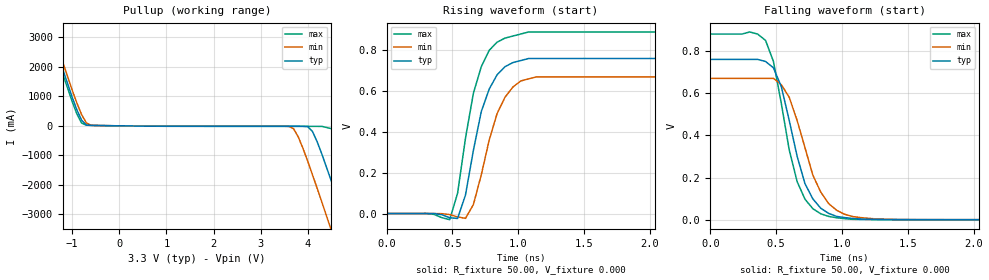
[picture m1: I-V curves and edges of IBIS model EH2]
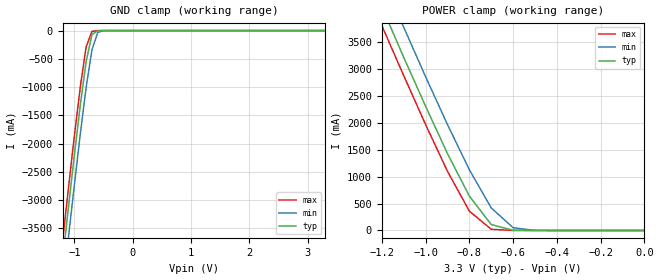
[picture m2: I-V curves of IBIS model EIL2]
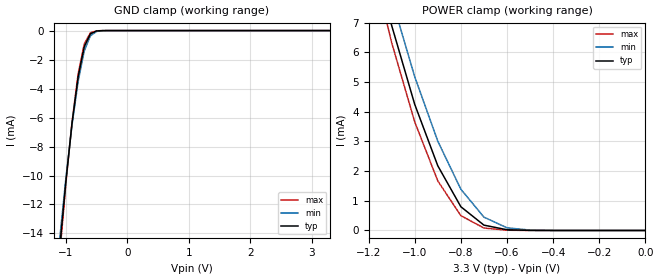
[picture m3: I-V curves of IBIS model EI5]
|   * 932s801a.ibs * IBIS 2.1 Model file
| Rev History
| Rev No.   Description
| 1.0   Initial release with Updated Parasitic Parameters
[IBIS Ver]   2.1
[Comment char]  |_char
[File name]   932s801a.ibs
[Date]   May 19, 2004
[File Rev]   1.0
[Source]   Originated at Integrated Circuit Systems, Inc.
[Disclaimer] (C) Copyright Integrated Circuit Systems, Inc. 2004
   All rights reserved
ICS hereby grants the user of this IBIS model a non-exclusive,
nontransferable license to use this IBIS model under the following terms.
Before using this IBIS model, the user should read this license.
If the user does not accept these terms,  the IBIS model should be
returned to ICS within 30 days.
   The user is granted this license only to use the IBIS model and
is not granted rights to sell, load, rent, lease or license the IBIS
model in whole or in part, or in modified form to anyone other than
user. User may modify the IBIS model to suit its specific
applications but rights to derivative works and such modifications
shall belong to ICS.
   This IBIS model is provided on an "AS IS" basis and ICS makes
absolutely no warranty with respect to the information contained
herein. ICS DISCLAIMS AND CUSTOMER WAIVES ALL WARRANTIES, EXPRESS
OR IMPLIED, INCLUDING WARRANTIES OF MERCHANTABILITY OR FITNESS FOR
A PARTICULAR PURPOSE. The entire risk as to quality and performance
is with the Customer. ACCORDINGLY, IN NO EVENT SHALL THE COMPANY BE
LIABLE FOR ANY DAMAGES, WHETHER IN CONTRACT OR TORT,INCLUDING ANY
LOST PROFITS OR OTHER INCIDENTAL, CONSEQUENTIAL, EXEMPLARY, OR
PUNITIVE DAMAGES ARISING OUT OF THE USE OR APPLICATION OF THE IBIS
model provided in this package. Further, ICS reserves the right to
make changes without notice to any product herein to improve
reliability, function, or design. ICS does not convey any license
under patent rights or any other intellectual property rights,
including those of third parties.
   ICS is not obligated to provide maintenance or support
for the licensed IBIS model.
|   COMPONENT: ICS932s801a
[Component]   ICS932s801a
[Manufacturer]  ICS
[Package]
| variable   typ   min   max
R_pkg   81.1m   62.2m   100.0m
L_pkg   6.7nH   4.9nH   8.5nH
C_pkg   0.53pF  0.21pF  0.85pF
[Pin]   signal_name   model_name   R_pin   L_pin   C_pin
  1   X1   EIX
  2   X2   EIX
  3   VDD48   POWER
  4   M48_0   YO39
  5   M48_1   YO39
  6   GND   GND
  7   SCLK   EI8
  8   SDATA   EIOD1
  9   VDDHTT   POWER
  10   HTTCLK0   FIO2
  11   HTTCLK1   FIO2
  12   HTTCLK2   FIO2
  13   HTTCLK3   FIO2
  14   GND   GND
  15   VDDPCI   POWER
  16   PCI0   FIO2
  17   PCI1   FIO2
  18   PCI2   FIO2
  19   PCI3   FIO2
  20   GND   GND
  21   PDB   EI5
  22   VDDA   POWER
  23   VSSA   GND
  24   IREF   EI5
  25   SRCCLKC0   EH2
  26   SRCCLKT0   EH2
  27   VDDSRC   POWER
  28   GND   GND
  29   SPREAD_EN   EI5
  30   CPU3B   DO10
  31   CPU3   DO10
  32   VSSCPU   GND
  33   VDDCPU   POWER
  34   CPU2B   DO10
  35   CPU2   DO10
  36   VSSCPU   GND
  37   VDDCPU   POWER
  38   CPU1B   DO10
  39   CPU1   DO10
  40   VSSCPU   GND
  41   VDDCPU   POWER
  42   CPU0B   DO10
  43   CPU0   DO10
  44   GND   GND
  45   FS2   EIL2
  46   FS1_REF1   EIO20
  47   FS0_REF0   EIO20
  48   VDDREF   POWER
|* Either 3.3V or 2.5V
|** All model are simulated with typical corner process
[Diff Pin]   inv_pin   vdiff   tdelay_typ
14   15   NA   NA
17   18   NA   NA
21   22   NA   NA
23   24   NA   NA
26   27   NA   NA
31   30   NA   NA
33   32   NA   NA
36   35   NA   NA
42   41   NA   NA
45   44   NA   NA
| Models and submodels in the file (10): EH2 (Open_source), EIL2 (Input), EI5 (Input), EI8 (Input), EIOD1 (I/O_open_drain), EIX (Input), DO10 (Output), FIO2 (I/O), EIO20 (I/O), YO39 (Output)
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|   Model EH2
[Model]   EH2
Model_type   Open_source
Polarity   Inverting
C_comp   5.50pF   5.00pF   6.00pF
[Temperature Range]   27.00   70.00   0.000
[Voltage Range]   3.30V   3.00V   3.70V
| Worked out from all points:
|   slope of the pullup table from 0 to 0.495 V, typ, clamps not added: 56.2 ohm
|   rising waveform, R_fixture 50.00, V_fixture 0.000: 20-80 % time 162ps typ, 178ps min, 159ps max; typ from 0 V to 0.76 V
|   falling waveform, R_fixture 50.00, V_fixture 0.000: 20-80 % time 187ps typ, 213ps min, 169ps max; typ from 0.76 V to 0 V
[Pullup]
| voltage   I(typ)   I(min)   I(max)
-3.3V     12.3A      12.52A     12.16A
-1.7V     4.31A      4.55A      4.16A
-1.5V     3.33A      3.58A      3.17A
-900mV    540mA      770mA      400mA
-700mV    28.62mA    98.17mA    20.44mA
3.7V      -15.27mA   -98.54mA   -17.77mA
4.1V      -190mA     -1.66A     -17.8mA
4.5V      -1.87A     -3.54A     -94.68mA
4.7V      -2.82A     -4.51A     -810mA
4.9V      -3.78A     -5.48A     -1.72A
5.3V      -5.73A     -7.43A     -3.63A
6.6V      -12.13A    -13.84A    -10.01A
[Ramp]
| variable   typ   min   max
dV/dt_r   0.46/0.16n   0.40/0.17n   0.53/0.15n
dV/dt_f   0.45/0.18n   0.40/0.20n   0.53/0.17n
R_load = 50.00
[Rising Waveform]
R_fixture = 50.00
V_fixture = 0.000
V_fixture_min = 0.000
V_fixture_max = 0.000
| time   V(typ)   V(min)   V(max)
0s        0V         0V         0V
480ps     -20.65mV   -5.16mV    -30.15mV
540ps     -24.16mV   -16.59mV   100mV
600ps     91.23mV    -23.49mV   370mV
660ps     310mV      44.3mV     590mV
720ps     500mV      190mV      720mV
840ps     680mV      490mV      840mV
900ps     720mV      570mV      860mV
1.14ns    760mV      670mV      890mV
3ns       760mV      670mV      890mV
[Falling Waveform]
R_fixture = 50.00
V_fixture = 0.000
V_fixture_min = 0.000
V_fixture_max = 0.000
| time   V(typ)   V(min)   V(max)
0s        760mV      670mV      880mV
420ps     750mV      670mV      850mV
480ps     720mV      670mV      750mV
540ps     630mV      640mV      550mV
660ps     300mV      470mV      180mV
720ps     170mV      340mV      96.56mV
840ps     53.88mV    130mV      27.79mV
960ps     15.52mV    44.77mV    8.96mV
1.14ns    3.29mV     9.98mV     1.1mV
3ns       2.98uV     6.39uV     2.37uV
|   Model EIL2
[Model]   EIL2
Model_type   Input
Polarity   Inverting
Enable   Active-High
Vinl =   0.80V
Vinh =   2.00V
C_comp   5.50pF   5.00pF   6.00pF
[Temperature Range]   27.00   70.00   0.000
[Voltage Range]   3.30V   3.00V   3.70V
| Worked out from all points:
|   GND clamp passes 1 mA (typ) near -0.54 V on its own axis
|   POWER clamp passes 1 mA (typ) near -0.53 V on its own axis
[GND_clamp]
| voltage   I(typ)   I(min)   I(max)
-3.3V     -24.56A    -25.06A    -24.25A
-1.2V     -4.03A     -4.57A     -3.69A
-1.1V     -3.1A      -3.63A     -2.76A
-1V       -2.19A     -2.72A     -1.85A
-900mV    -1.32A     -1.83A     -1A
-800mV    -550mA     -1.01A     -290mA
-700mV    -72.12mA   -340mA     -14.48mA
-600mV    -2.27mA    -32.49mA   -430uA
-500mV    -86.13uA   -1.31mA    -27.26uA
3.3V      71.49pA    2.77uA     48.86pA
[POWER_clamp]
| voltage   I(typ)   I(min)   I(max)
-3.3V     24.7A      25.22A     24.38A
-1.2V     4.16A      4.71A      3.81A
-1.1V     3.22A      3.78A      2.88A
-1V       2.31A      2.86A      1.97A
-900mV    1.43A      1.97A      1.1A
-800mV    640mA      1.13A      360mA
-700mV    110mA      420mA      22.36mA
-600mV    3.4mA      51.05mA    380uA
-500mV    80.25uA    2.14mA     6.04uA
0V        71.49pA    320pA      74.54pA
|   Model EI5
[Model]   EI5
Model_type   Input
Polarity   Non-Inverting
Vinl =   0.80V
Vinh =   2.00V
C_comp   5.50pF   5.00pF   6.00pF
[Temperature Range]   27.00   70.00   0.000
[Voltage Range]   3.30V   3.00V   3.70V
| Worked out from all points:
|   GND clamp passes 1 mA (typ) near -0.69 V on its own axis
|   POWER clamp passes 1 mA (typ) near -0.81 V on its own axis
[GND_clamp]
| voltage   I(typ)   I(min)   I(max)
-3.3V     -140mA     -130mA     -150mA
-1.1V     -15.03mA   -14.4mA    -15.5mA
-1V       -10.44mA   -10.23mA   -10.61mA
-900mV    -6.42mA    -6.53mA    -6.34mA
-800mV    -3.2mA     -3.51mA    -2.98mA
-700mV    -1.11mA    -1.4mA     -910uA
-600mV    -220uA     -360uA     -150uA
-500mV    -27.68uA   -59.14uA   -15.29uA
-400mV    -2.43uA    -7.33uA    -1.01uA
3.3V      150pA      140nA      93.85pA
[POWER_clamp]
| voltage   I(typ)   I(min)   I(max)
-3.3V     150mA      140mA      150mA
-1.2V     10.05mA    10.86mA    9.56mA
-1.1V     6.91mA     7.82mA     6.33mA
-1V       4.25mA     5.18mA     3.66mA
-900mV    2.18mA     3.01mA     1.67mA
-800mV    800uA      1.39mA     500uA
-700mV    180uA      450uA      82.19uA
-600mV    23.89uA    89.39uA    8.44uA
-500mV    2.38uA     12.85uA    610nA
0V        150pA      1.12nA     140pA
